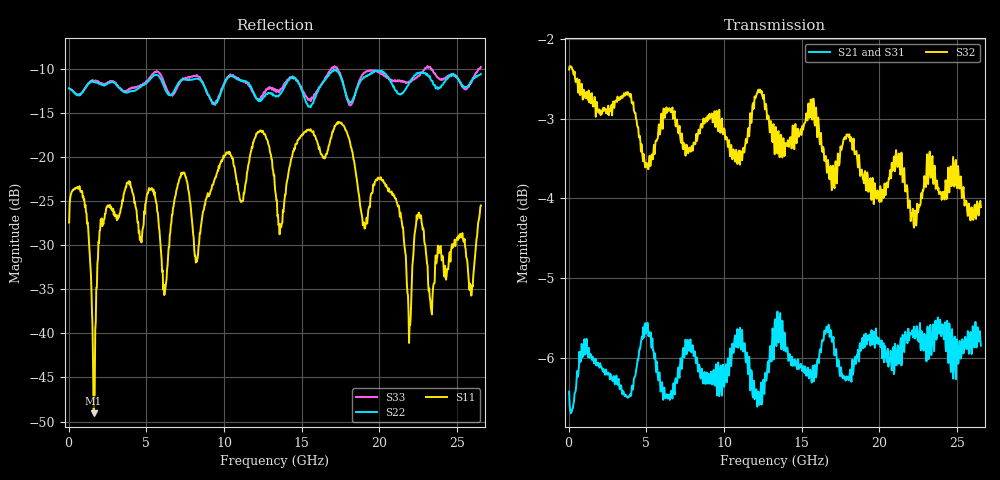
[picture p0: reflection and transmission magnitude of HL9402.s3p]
! 2/9/2021 10:31:58 AM
! H:\PRODUCTION_DATA\TEMP_S3P.S3P
! CHANNEL.1
! TR.MEASUREMENT
! CORRECTED.DATA
# GHZ S RI R 50.0
! FREQ.GHZ  S11RE  S11IM  S12RE  S12IM  S13RE  S13IM
!  S21RE  S21IM  S22RE  S22IM  S23RE  S23IM
!  S31RE  S31IM  S32RE  S32IM  S33RE  S33IM
!; PortSelection: Port_123
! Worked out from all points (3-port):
!   758 points, 35 MHz to 26.53 GHz, reference 50 ohm
!   strongest paths, dB at 35 MHz, 6.65 GHz, 13.3 GHz, 19.91 GHz, 26.53 GHz:
!     S32: -2.4, -2.9, -3.2, -3.9, -4.1
!     S21: -6.4, -6.5, -5.5, -5.8, -5.8
!     S31: -6.4, -6.3, -5.8, -5.7, -5.6
!   lowest |S11| = -49.1 dB at 1.61 GHz (marker M1), VSWR 1.01, Z = 49.8 - j0.302 ohm
!   |S11| at or under -10 dB: start of sweep to end of sweep
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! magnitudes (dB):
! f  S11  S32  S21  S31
! 35 MHz  -27.5  -2.4  -6.4  -6.4
! 1.05 GHz  -25.7  -2.7  -6.0  -5.9
! 1.61 GHz  -49.1  -2.8  -6.0  -6.1
! 2.03 GHz  -28.3  -2.9  -6.1  -6.0
! 3.85 GHz  -23.0  -2.7  -6.5  -6.5
! 6.195 GHz  -35.4  -3.0  -6.4  -6.5
! 13.3 GHz  -23.9  -3.2  -5.5  -5.8
! 17.61 GHz  -16.4  -3.3  -6.2  -6.2
! 21.95 GHz  -38.6  -4.0  -5.7  -6.0
! 26.53 GHz  -25.5  -4.1  -5.8  -5.6
